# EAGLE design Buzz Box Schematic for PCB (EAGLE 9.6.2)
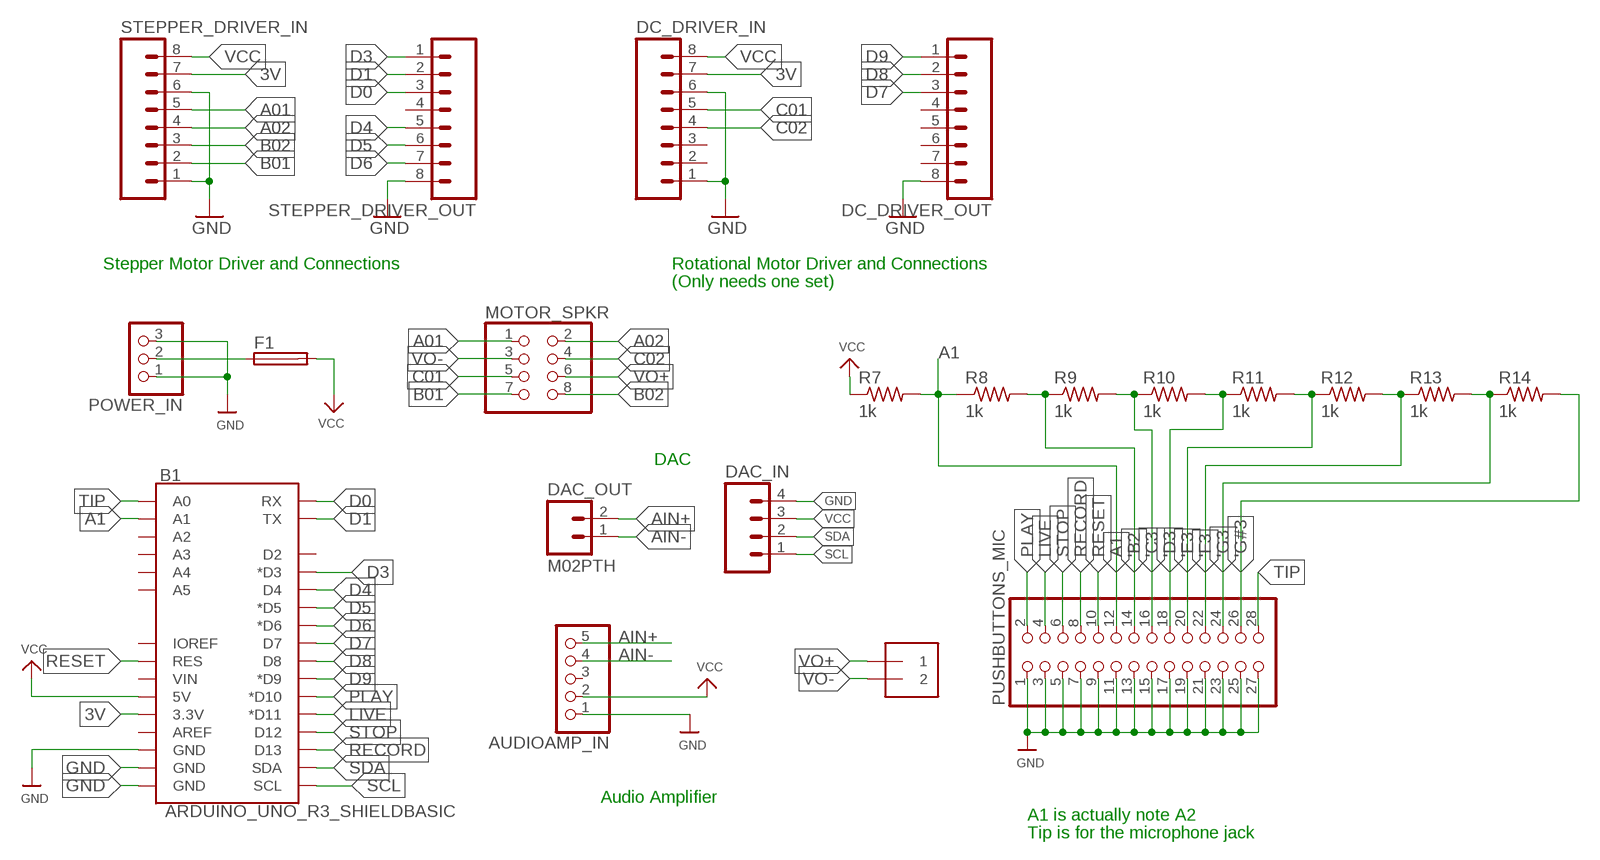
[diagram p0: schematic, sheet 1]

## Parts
AUDIOAMP_IN  HEADER-1X570MIL  [1X05_ROUND_70]
AUDIOAMP_OUT  TERMBLOCK_1X2  [TERMBLOCK_1X2-3.5MM]
B1  ARDUINO_UNO_R3_SHIELDBASIC  [UNO_R3_SHIELD]
DAC_IN  M04PTH  [1X04]
DAC_OUT  M02PTH  [1X02]
DC_DRIVER_IN  M08PTH  [1X08]
DC_DRIVER_OUT  M08PTH  [1X08]
F1  19560  [19560]
MOTOR_SPKR  PINHD-2X4  [2X04]
POWER_IN  PINHD-1X3  [1X03]
PUSHBUTTONS_MIC  PINHD-2X14  [2X14]
R7  1k  R-US_0207/10  [0207/10]
R8  1k  R-US_0207/10  [0207/10]
R9  1k  R-US_0207/10  [0207/10]
R10  1k  R-US_0207/10  [0207/10]
R11  1k  R-US_0207/10  [0207/10]
R12  1k  R-US_0207/10  [0207/10]
R13  1k  R-US_0207/10  [0207/10]
R14  1k  R-US_0207/10  [0207/10]
STEPPER_DRIVER_IN  M08PTH  [1X08]
STEPPER_DRIVER_OUT  M08PTH  [1X08]

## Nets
3V: B1.3.3V DC_DRIVER_IN.7 STEPPER_DRIVER_IN.7
5VOLTS: F1.1 POWER_IN.2
'B2: PUSHBUTTONS_MIC.14 R8.2 R9.1
'C3: PUSHBUTTONS_MIC.16 R9.2 R10.1
'D3: PUSHBUTTONS_MIC.18 R10.2 R11.1
'E3: PUSHBUTTONS_MIC.20 R11.2 R12.1
'F3: PUSHBUTTONS_MIC.22 R12.2 R13.1
'G3: PUSHBUTTONS_MIC.24 R13.2 R14.1
'G#3: PUSHBUTTONS_MIC.26 R14.2
A1: B1.A1 PUSHBUTTONS_MIC.12 R7.2 R8.1
A01: MOTOR_SPKR.1 STEPPER_DRIVER_IN.5
A02: MOTOR_SPKR.2 STEPPER_DRIVER_IN.4
AIN+: AUDIOAMP_IN.5 DAC_OUT.2
AIN-: AUDIOAMP_IN.4 DAC_OUT.1
B01: MOTOR_SPKR.7 STEPPER_DRIVER_IN.2
B02: MOTOR_SPKR.8 STEPPER_DRIVER_IN.3
C01: DC_DRIVER_IN.5 MOTOR_SPKR.5
C02: DC_DRIVER_IN.4 MOTOR_SPKR.4
D0: B1.RX STEPPER_DRIVER_OUT.3
D1: B1.TX STEPPER_DRIVER_OUT.2
D3: B1.D3(*D3) STEPPER_DRIVER_OUT.1
D4: B1.D4 STEPPER_DRIVER_OUT.5
D5: B1.D5(*D5) STEPPER_DRIVER_OUT.6
D6: B1.D6(*D6) STEPPER_DRIVER_OUT.7
D7: B1.D7 DC_DRIVER_OUT.3
D8: B1.D8 DC_DRIVER_OUT.2
D9: B1.D9(*D9) DC_DRIVER_OUT.1
GND: AUDIOAMP_IN.1 B1.GND@0(GND) B1.GND@1(GND) B1.GND@2(GND) DAC_IN.4 DC_DRIVER_IN.1 DC_DRIVER_IN.6 DC_DRIVER_OUT.8 POWER_IN.1 POWER_IN.3 PUSHBUTTONS_MIC.1 PUSHBUTTONS_MIC.3 PUSHBUTTONS_MIC.5 PUSHBUTTONS_MIC.7 PUSHBUTTONS_MIC.9 PUSHBUTTONS_MIC.11 PUSHBUTTONS_MIC.13 PUSHBUTTONS_MIC.15 PUSHBUTTONS_MIC.17 PUSHBUTTONS_MIC.19 PUSHBUTTONS_MIC.21 PUSHBUTTONS_MIC.23 PUSHBUTTONS_MIC.25 PUSHBUTTONS_MIC.27 STEPPER_DRIVER_IN.1 STEPPER_DRIVER_IN.6 STEPPER_DRIVER_OUT.8
LIVE: B1.D11(*D11) PUSHBUTTONS_MIC.4
PLAY: B1.D10(*D10) PUSHBUTTONS_MIC.2
RECORD: B1.D13 PUSHBUTTONS_MIC.8
RESET: B1.RES PUSHBUTTONS_MIC.10
SCL: B1.SCL DAC_IN.1
SDA: B1.SDA DAC_IN.2
STOP: B1.D12 PUSHBUTTONS_MIC.6
TIP: B1.A0 PUSHBUTTONS_MIC.28
VCC: AUDIOAMP_IN.2 B1.5V DAC_IN.3 DC_DRIVER_IN.8 F1.2 R7.1 STEPPER_DRIVER_IN.8
VO+: AUDIOAMP_OUT.1 MOTOR_SPKR.6
VO-: AUDIOAMP_OUT.2 MOTOR_SPKR.3
Unconnected: AUDIOAMP_IN.3 B1.A2 B1.A3 B1.A4 B1.A5 B1.AREF B1.D2 B1.IOREF B1.VIN DC_DRIVER_IN.2 DC_DRIVER_IN.3 DC_DRIVER_OUT.4 DC_DRIVER_OUT.5 DC_DRIVER_OUT.6 DC_DRIVER_OUT.7 STEPPER_DRIVER_OUT.4

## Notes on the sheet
- Stepper Motor Driver and Connections | Rotational Motor Driver and Connections
- (Only needs one set)
- DAC
- Audio Amplifier
- A1 is actually note A2
- Tip is for the microphone jack

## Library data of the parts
AUDIOAMP_IN = microbuilder:HEADER-1X5: PIN HEADER
AUDIOAMP_OUT = microbuilder:TERMBLOCK_1X2: 3.5mm Terminal block
B1 = SparkFun-Boards:ARDUINO_UNO_R3_SHIELD: Arduino R3 Shield Footprint Shield form compatible with the Arduino Uno R3. SparkFun Products: MG2639 Cellular Shield MIDI Shield R3 Stackable Headers Kit
DAC_IN = SparkFun-Connectors:M04: Header 4 Standard 4-pin 0.1" header. Use with straight break away headers (SKU : PRT-00116), right angle break away headers (PRT-00553), swiss pins (PRT-00743), machine pins (PRT-00117), and female headers (PRT-00115). Molex polarized connector foot print use with SKU : PRT-08231 with associated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
DAC_OUT = SparkFun-Connectors:M02: Standard 2-pin 0.1" header. Use with
DC_DRIVER_IN DC_DRIVER_OUT STEPPER_DRIVER_IN STEPPER_DRIVER_OUT = Testing:M08: Header 8 Standard 8-pin 0.1" header. Use with straight break away headers (SKU : PRT-00116), right angle break away headers (PRT-00553), swiss pins (PRT-00743), machine pins (PRT-00117), and female headers (PRT-00115).
F1 = fuse:19560: FUSE HOLDER; MPN: 56000001009; OC_FARNELL: 1185363; OC_NEWARK: 15P8392
MOTOR_SPKR = adafruit:PINHD-2X4: PIN HEADER
POWER_IN = adafruit:PINHD-1X3: PIN HEADER
PUSHBUTTONS_MIC = adafruit:PINHD-2X14: PIN HEADER
R7-R14 = rcl:R-US_: RESISTOR, American symbol; SPICEPREFIX: R

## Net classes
0 default: width 0.305 mm, drill 0.508 mm, clearance 0.254 mm

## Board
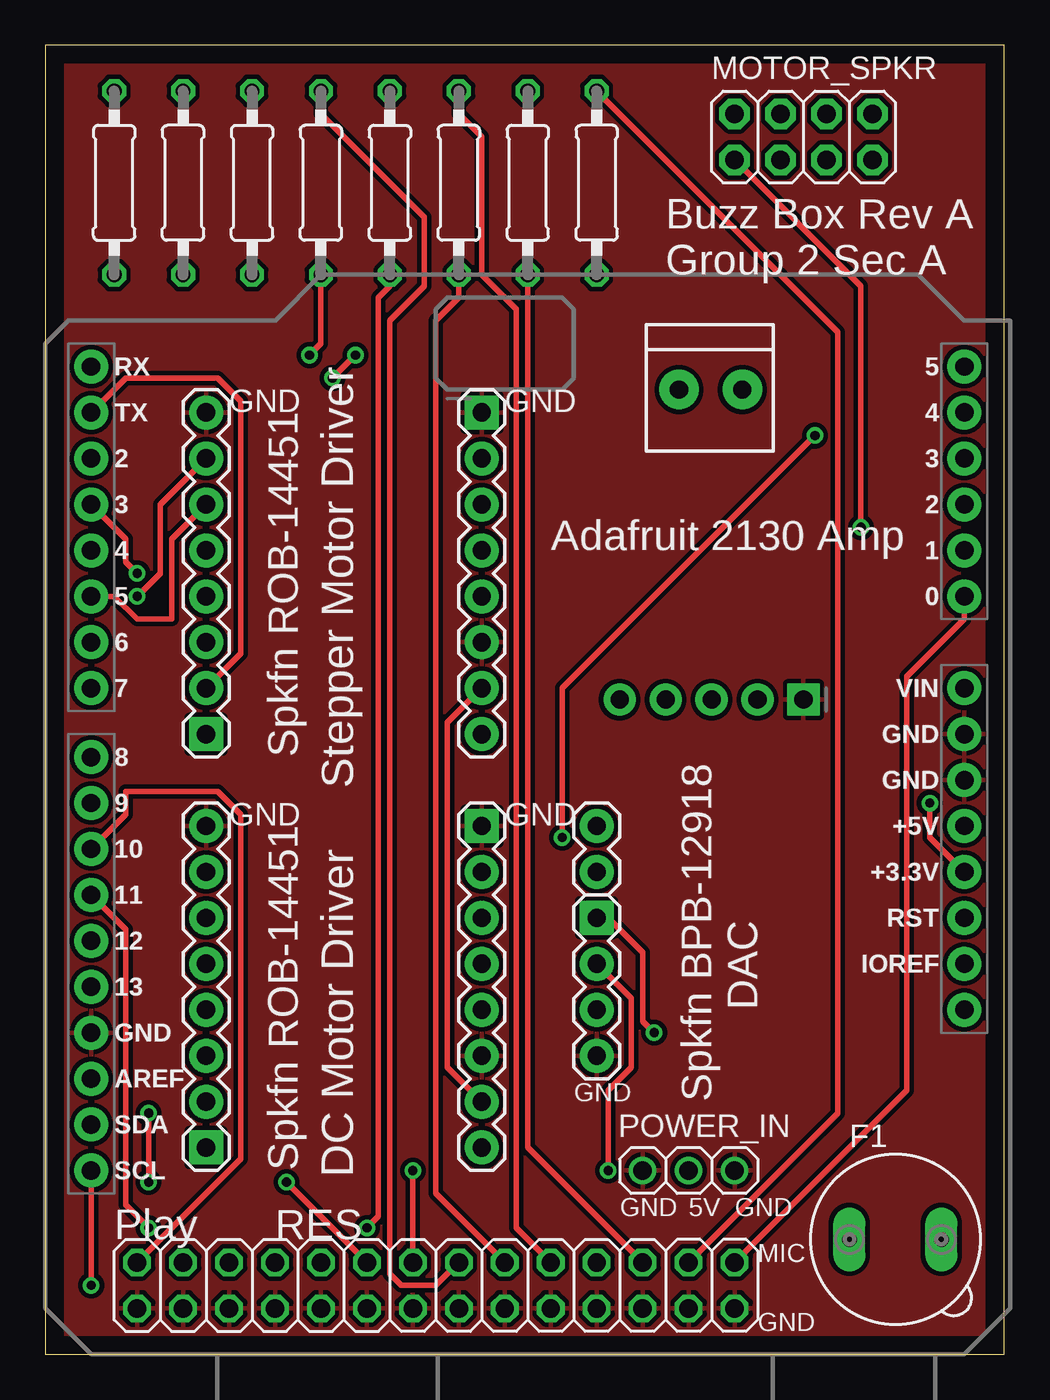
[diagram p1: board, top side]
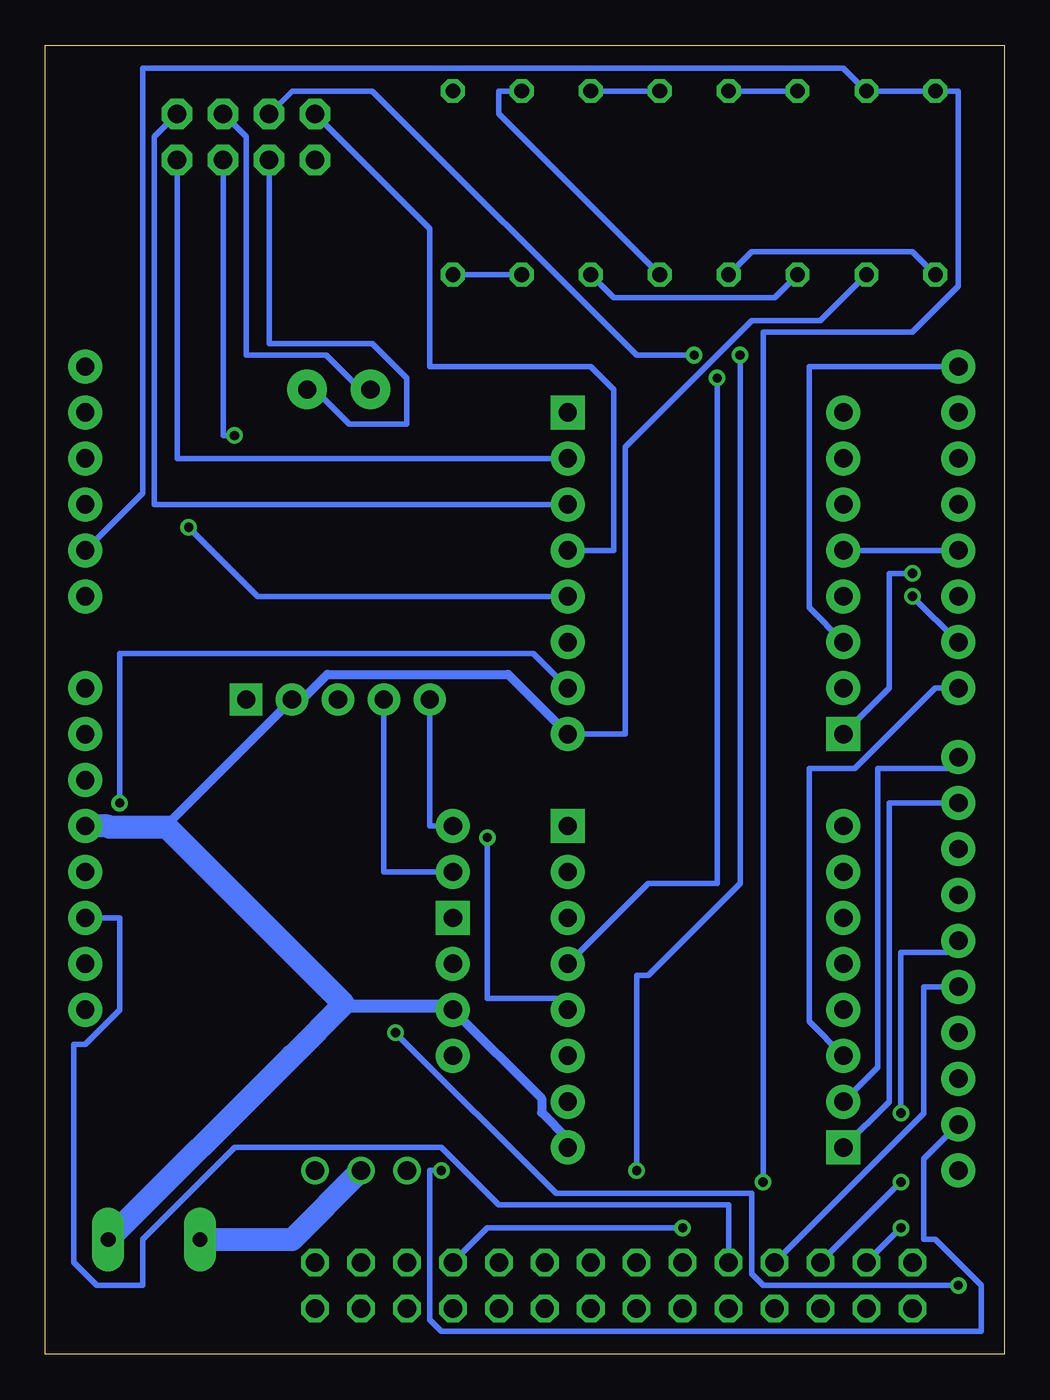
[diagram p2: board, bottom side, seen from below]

Size 53.01 x 72.38 mm. Coordinates in mm from the lower left corner, seen from the top.
Outline: 0,0 53.01,0 53.01,72.38 0,72.38 0,0
Copper layers (1*16): Top 0.035mm / dielectric 1.5mm / Bottom 0.035mm
Design rules "default": minimum track width 6mil, minimum drill 0.35mm, track to track 6mil, track to pad 6mil, pad to pad 6mil, via to via 6mil, smd to smd 6mil, copper to edge 40mil, drill to drill 6mil, minimum pad ring 10mil, minimum via ring 8mil, stop-mask expansion 4mil, vias tented up to drill 0mil, thermal gap 10mil

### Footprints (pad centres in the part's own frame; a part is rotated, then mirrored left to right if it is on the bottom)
1X05_ROUND_70 = drill 1 pad 1.778 square: 1 -5.08,0 | drill 1 pad 1.778: 2 -2.54,0; 3 0,0; 4 2.54,0; 5 5.08,0
TERMBLOCK_1X2-3.5MM = drill 1 pad 2.184: 1 1.8,0; 2 -1.7,0
UNO_R3_SHIELD = drill 1.016 pad 1.88: 3.3V 24.13,-2.54; 5V 24.13,0; A0 24.13,12.7; A1 24.13,15.24; A2 24.13,17.78; A3 24.13,20.32; A4 24.13,22.86; A5 24.13,25.4; AREF -24.13,-13.97; D2 -24.13,20.32; D3 -24.13,17.78; D4 -24.13,15.24; D5 -24.13,12.7; D6 -24.13,10.16; D7 -24.13,7.62; D8 -24.13,3.81; D9 -24.13,1.27; D10 -24.13,-1.27; D11 -24.13,-3.81; D12 -24.13,-6.35; D13 -24.13,-8.89; GND@0 24.13,2.54; GND@1 24.13,5.08; GND@2 -24.13,-11.43; IOREF 24.13,-7.62; NC 24.13,-10.16; RES 24.13,-5.08; RX -24.13,25.4; SCL -24.13,-19.05; SDA -24.13,-16.51; TX -24.13,22.86; VIN 24.13,7.62
1X04 = drill 1.016 pad 1.88 square: 1 0,0 | drill 1.016 pad 1.88: 2 2.54,0; 3 5.08,0; 4 7.62,0
1X02 = drill 1.016 pad 1.88: 1 0,0; 2 2.54,0
1X08 = drill 1.016 pad 1.88 square: 1 0,0 | drill 1.016 pad 1.88: 2 2.54,0; 3 5.08,0; 4 7.62,0; 5 10.16,0; 6 12.7,0; 7 15.24,0; 8 17.78,0
19560 = drill 0.813 pad 1.778 long: 1 -2.54,0; 2 2.54,0
2X04 = drill 1.016 pad 1.676 octagon: 1 -3.81,-1.27; 2 -3.81,1.27; 3 -1.27,-1.27; 4 -1.27,1.27; 5 1.27,-1.27; 6 1.27,1.27; 7 3.81,-1.27; 8 3.81,1.27
1X03 = drill 1.016: 1 -2.54,0; 2 0,0; 3 2.54,0
2X14 = drill 1.016 octagon: 1 -16.51,-1.27; 2 -16.51,1.27; 3 -13.97,-1.27; 4 -13.97,1.27; 5 -11.43,-1.27; 6 -11.43,1.27; 7 -8.89,-1.27; 8 -8.89,1.27; 9 -6.35,-1.27; 10 -6.35,1.27; 11 -3.81,-1.27; 12 -3.81,1.27; 13 -1.27,-1.27; 14 -1.27,1.27; 15 1.27,-1.27; 16 1.27,1.27; 17 3.81,-1.27; 18 3.81,1.27; 19 6.35,-1.27; 20 6.35,1.27; 21 8.89,-1.27; 22 8.89,1.27; 23 11.43,-1.27; 24 11.43,1.27; 25 13.97,-1.27; 26 13.97,1.27; 27 16.51,-1.27; 28 16.51,1.27
0207/10 = drill 0.813 octagon: 1 -5.08,0; 2 5.08,0

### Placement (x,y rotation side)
AUDIOAMP_IN  36.83,36.2 180 top
AUDIOAMP_OUT  36.83,53.34 180 top
B1  26.67,29.21 0 top
DAC_IN  30.48,24.13 270 top
DAC_OUT  30.48,26.67 90 top
DC_DRIVER_IN  24.13,29.21 270 top
DC_DRIVER_OUT  8.89,11.43 90 top
F1  46.99,6.35 0 top
MOTOR_SPKR  41.91,67.31 0 top
POWER_IN  35.56,10.16 0 top
PUSHBUTTONS_MIC  21.59,3.81 0 top
R7  7.62,64.77 90 top
R8  3.81,64.77 270 top
R9  15.24,64.77 90 top
R10  11.43,64.77 270 top
R11  22.86,64.77 90 top
R12  19.05,64.77 270 top
R13  26.67,64.77 270 top
R14  30.48,64.77 90 top
STEPPER_DRIVER_IN  24.13,52.07 270 top
STEPPER_DRIVER_OUT  8.89,34.29 90 top

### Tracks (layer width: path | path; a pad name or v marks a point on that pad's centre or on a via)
3V  (via drill 0.51)
  Top 0.305: DC_DRIVER_IN.7 22.23,15.88 22.23,34.92 23.5,36.2 24.13,36.2 STEPPER_DRIVER_IN.7 | B1.3.3V 48.9,28.57 v48.9,30.48
  Bottom 0.305: v48.9,30.48 48.9,38.73 26.04,38.73 STEPPER_DRIVER_IN.7
5VOLTS
  Bottom 1.27: F1.1 39.37,6.35 POWER_IN.2
'B2  (via drill 0.51)
  Top 0.305: v20.32,10.16 PUSHBUTTONS_MIC.14 | v14.61,55.24 15.24,55.88 R9.1
  Bottom 0.305: R8.2 5.08,60.96 13.97,60.96 R9.1 | v20.32,10.16 20.32,20.95 19.68,20.95 14.61,26.04 v14.61,55.24
'C3
  Top 0.305: PUSHBUTTONS_MIC.16 21.59,3.81 19.68,3.81 19.05,4.45 19.05,57.15 20.95,59.05 20.95,62.87 15.24,68.58 R9.2
  Bottom 0.305: R9.2 R10.1
'D3
  Top 0.305: PUSHBUTTONS_MIC.18 21.59,8.89 21.59,57.15 22.86,58.42 R11.1
  Bottom 0.305: R10.2 12.7,58.42 21.59,58.42 R11.1
'E3
  Top 0.305: PUSHBUTTONS_MIC.20 26.04,6.99 26.04,57.78 24.13,59.69 24.13,67.31 22.86,68.58 R11.2
  Bottom 0.305: R11.2 R12.1
'F3  (via drill 0.51)
  Top 0.305: v17.78,6.99 18.41,7.62 18.41,58.42 19.05,59.05 R12.2
  Bottom 0.305: R12.2 27.94,68.58 27.94,69.85 R13.1 | PUSHBUTTONS_MIC.22 28.57,6.99 v17.78,6.99
'G3
  Top 0.305: PUSHBUTTONS_MIC.24 26.67,11.43 R13.2
  Bottom 0.305: R14.1 R13.2
'G#3
  Top 0.305: R14.2 43.81,56.52 43.81,13.34 PUSHBUTTONS_MIC.26
A1  (via drill 0.51)
  Top 0.305: v13.34,9.53 PUSHBUTTONS_MIC.12
  Bottom 0.305: v13.34,9.53 13.34,56.52 5.08,56.52 2.54,59.05 2.54,69.85 R8.1 R7.2 8.89,71.12 47.62,71.12 47.62,47.62 B1.A1
A01  (via drill 0.51)
  Top 0.305: MOTOR_SPKR.1 45.09,59.05 v45.09,45.72
  Bottom 0.305: v45.09,45.72 41.27,41.91 STEPPER_DRIVER_IN.5
A02
  Bottom 0.305: MOTOR_SPKR.2 31.75,62.23 31.75,54.61 22.86,54.61 21.59,53.34 21.59,44.45 STEPPER_DRIVER_IN.4
AIN+
  Bottom 0.305: AUDIOAMP_IN.5 31.75,29.21 DAC_OUT.2
AIN-
  Bottom 0.305: AUDIOAMP_IN.4 34.29,26.67 DAC_OUT.1
B01
  Bottom 0.305: MOTOR_SPKR.7 45.72,49.53 STEPPER_DRIVER_IN.2
B02
  Bottom 0.305: MOTOR_SPKR.8 46.99,67.31 46.99,46.99 STEPPER_DRIVER_IN.3
C01  (via drill 0.51)
  Top 0.305: v42.55,50.8 28.57,36.83 v28.57,28.57
  Bottom 0.305: MOTOR_SPKR.5 43.18,50.8 v42.55,50.8 | v28.57,28.57 28.57,19.68 24.77,19.68 DC_DRIVER_IN.5
C02  (via drill 0.51)
  Top 0.305: v15.88,53.98 v17.14,55.24
  Bottom 0.305: MOTOR_SPKR.4 39.37,69.85 34.92,69.85 20.32,55.24 v17.14,55.24 | v15.88,53.98 15.88,26.04 19.68,26.04 DC_DRIVER_IN.4
D0
  Bottom 0.305: STEPPER_DRIVER_OUT.3 10.79,41.27 10.79,54.61 B1.RX
D1
  Top 0.305: STEPPER_DRIVER_OUT.2 10.79,38.73 10.79,52.7 9.53,53.98 4.45,53.98 3.17,52.7 2.54,52.7 B1.TX
D3  (via drill 0.51)
  Top 0.305: v5.08,43.18 4.45,43.81 4.45,45.09 3.17,46.35 2.54,46.35 B1.D3
  Bottom 0.305: STEPPER_DRIVER_OUT.1 6.35,36.83 6.35,43.18 v5.08,43.18
D4
  Bottom 0.305: STEPPER_DRIVER_OUT.5 B1.D4
D5
  Top 0.305: B1.D5 3.81,41.91 5.08,40.64 6.99,40.64 6.99,45.09 8.26,46.35 8.89,46.35 STEPPER_DRIVER_OUT.6
D6  (via drill 0.51)
  Top 0.305: v5.08,41.91 6.35,43.18 6.35,46.99 8.26,48.9 8.89,48.9 STEPPER_DRIVER_OUT.7
  Bottom 0.305: v5.08,41.91 B1.D6
D7
  Bottom 0.305: DC_DRIVER_OUT.3 10.79,18.41 10.79,32.38 8.26,32.38 3.81,36.83 B1.D7
D8
  Bottom 0.305: DC_DRIVER_OUT.2 6.99,15.88 6.99,32.38 3.17,32.38 B1.D8
D9
  Bottom 0.305: DC_DRIVER_OUT.1 6.35,13.97 6.35,30.48 B1.D9
GND
  pour Top: 0,0 0,72.39 53.34,72.39 53.34,0
LIVE  (via drill 0.51)
  Top 0.305: v5.71,6.99 4.45,8.26 4.45,23.5 3.17,24.77 2.54,24.77 B1.D11
  Bottom 0.305: v5.71,6.99 PUSHBUTTONS_MIC.4
PLAY
  Top 0.305: PUSHBUTTONS_MIC.2 10.79,10.79 10.79,29.84 9.53,31.11 4.45,31.11 4.45,29.84 3.17,28.57 2.54,28.57 B1.D10
RECORD
  Bottom 0.305: PUSHBUTTONS_MIC.8 4.45,13.34 4.45,20.32 B1.D13
RESET
  Bottom 0.305: PUSHBUTTONS_MIC.10 15.24,8.26 27.94,8.26 31.11,11.43 42.55,11.43 47.62,6.35 47.62,3.81 50.16,3.81 51.44,5.08 51.44,17.14 50.8,17.14 48.9,19.05 48.9,24.13 B1.RES
SCL  (via drill 0.51)
  Top 0.305: v2.54,3.81 B1.SCL | v33.66,17.78 33.02,18.41 33.02,22.23 31.11,24.13 DAC_IN.1
  Bottom 0.305: v2.54,3.81 13.34,3.81 13.97,4.45 13.97,8.89 24.77,8.89 v33.66,17.78
SDA  (via drill 0.51)
  Top 0.305: v31.11,10.16 31.11,14.61 32.38,15.88 32.38,19.68 31.11,20.95 30.48,20.95 DAC_IN.2
  Bottom 0.305: B1.SDA 4.45,10.79 4.45,6.35 3.81,6.35 1.27,3.81 1.27,1.27 31.11,1.27 31.75,1.91 31.75,10.16 v31.11,10.16
STOP  (via drill 0.51)
  Top 0.305: v5.71,13.34 v5.71,9.53
  Bottom 0.305: v5.71,9.53 PUSHBUTTONS_MIC.6 | v5.71,13.34 5.71,22.23 3.17,22.23 B1.D12
TIP
  Top 0.305: PUSHBUTTONS_MIC.28 47.62,14.61 47.62,37.47 50.8,40.64 B1.A0
VCC
  Bottom 0.305: R7.1 10.16,57.15 13.97,57.15 20.95,50.16 20.95,34.29 STEPPER_DRIVER_IN.8 | 46.35,29.21 46.04,29.53 | B1.5V 46.35,29.21 | 39.37,16.51 36.83,19.05 36.2,19.05 | DAC_IN.3 36.2,19.05 | 36.2,19.05 36.51,19.37 46.35,29.21
  Bottom 0.508: 36.51,19.37 30.8,19.37 DAC_IN.3 25.58,14.15 25.58,13.37 24.13,11.92 DC_DRIVER_IN.8 | 46.04,29.53 AUDIOAMP_IN.2 38.81,36.2 37.41,37.59 27.43,37.59 STEPPER_DRIVER_IN.8
  Bottom 1.27: F1.2 39.37,16.51 36.51,19.37 46.28,29.13 49.45,29.13 49.53,29.21 B1.5V
VO+
  Bottom 0.305: MOTOR_SPKR.6 41.91,67.31 41.91,55.24 37.47,55.24 35.56,53.34 AUDIOAMP_OUT.1
VO-
  Bottom 0.305: MOTOR_SPKR.3 40.64,55.88 34.92,55.88 33.02,53.98 33.02,51.44 36.2,51.44 38.1,53.34 AUDIOAMP_OUT.2

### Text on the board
tPlace: Buzz Box Rev A | Group 2 Sec A | Adafruit 2130 Amp | Spkfn ROB-14451 | DAC | GND | Spkfn BPB-12918 | Spkfn ROB-14451 | GND | 5V | GND | Play | RES | MIC | GND
tNames: Stepper Motor Driver | GND | GND | GND | GND | DC Motor Driver

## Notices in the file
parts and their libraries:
SparkFun-Boards: Licensing: Creative Commons ShareAlike 4.0 International - https://creativecommons.org/licenses/by-sa/4.0
SparkFun-Connectors: Licensing: CC v3.0 Share-Alike You are welcome to use this library for commercial purposes.
